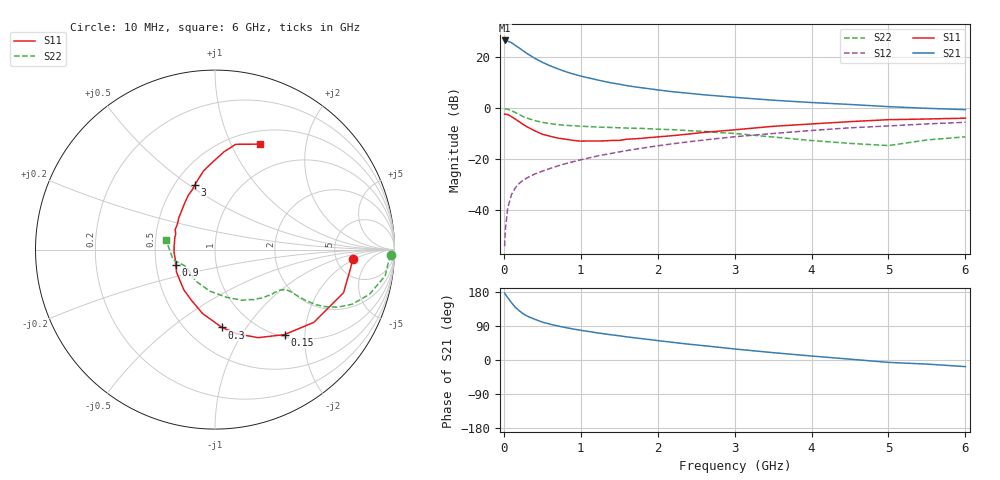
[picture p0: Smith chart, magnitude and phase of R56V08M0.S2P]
! SIEMENS Small Signal Semiconductors
! BFR183
! Si NPN RF Bipolar Junction Transistor in SOT23
! VCE = 6 V  IC = 8 mA
! Common Emitter S-Parameters:  May  1996
# GHz  S  MA  R  50
!  f  S11  S21  S12  S22
! GHz  MAG  ANG  MAG  ANG  MAG  ANG  MAG  ANG
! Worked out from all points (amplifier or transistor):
!   36 points, 10 MHz to 6 GHz, reference 50 ohm
!   highest |S21| = 26.5 dB at 10 MHz (marker M1)
!   |S21| within 3 dB of that: start of sweep to 202.4 MHz
!   unconditionally stable (mu >= 1): 884.2 MHz to 2.593 GHz
!   at 250 MHz: K = 0.54, MSG = 25.4 dB, |S12| = -28.2 dB
!   at 1.4 GHz: K = 1.05, MAG = 12.4 dB, |S12| = -17.7 dB
!   at 6 GHz: K = 0.88, MSG = 2.5 dB, |S12| = -5.5 dB
!   lowest NFmin = 1.30 dB at 450 MHz
!   S11 on the Smith chart (normalised r, x): 10 MHz: 7.21, -1.80; 150 MHz: 1.04, -1.58; 300 MHz: 0.73, -0.78; 900 MHz: 0.63, -0.11; 3 GHz: 0.63, +0.53; 6 GHz: 0.65, +1.30
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0.01  0.7694 -3.8  21.23 176.7  0.002 87.8  0.9827 -1.8
0.02  0.7628 -7.6  20.92 173.4  0.0043 87.5  0.9704 -3.6
0.05  0.7554 -18.5  20.54 164.7  0.011 81.1  0.9591 -8.8
0.1  0.6842 -36.3  19.14 151.0  0.0206 74.0  0.8955 -16.2
0.15  0.6118 -50.7  16.95 139.0  0.0279 67.2  0.8227 -21.7
0.2  0.5464 -63.9  15.12 129.9  0.0339 64.4  0.7533 -25.2
0.25  0.484 -75.6  13.36 122.1  0.0389 62.4  0.6906 -27.4
0.3  0.4353 -84.9  11.83 116.2  0.0433 61.2  0.6418 -28.6
0.4  0.3629 -101.0  9.558 107.6  0.0514 60.9  0.5759 -29.3
0.5  0.3104 -115.3  7.929 100.1  0.0587 61.4  0.53 -29.3
0.6  0.2838 -127.6  6.79 94.6  0.0661 61.8  0.4997 -29.2
0.7  0.261 -138.4  5.931 89.9  0.0743 63.0  0.4798 -29.0
0.9  0.2351 -158.6  4.69 81.9  0.09 62.9  0.4542 -29.4
1.1  0.2289 -175.5  3.934 75.3  0.1062 63.5  0.4377 -30.9
1.3  0.2295 169.3  3.36 69.2  0.1231 63.1  0.4247 -32.3
1.6  0.2481 153.4  2.772 61.0  0.1486 62.0  0.409 -35.7
2.2  0.2913 128.6  2.102 46.5  0.2021 57.9  0.3806 -44.7
3  0.3783 107.3  1.638 29.1  0.2767 50.1  0.3212 -61.6
3.5  0.4433 98.3  1.436 19.4  0.3207 44.3  0.2738 -76.3
4.5  0.5474 84.7  1.187 2.2  0.4144 32.4  0.2054 -121.9
5.5  0.6167 72.1  0.997 -10.8  0.4939 20.6  0.2399 -166.4
6  0.6392 66.9  0.941 -17.4  0.5314 12.8  0.2762 169.4
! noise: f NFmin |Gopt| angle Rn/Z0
0.45  1.3  0.17  43  0.21
0.9  1.35  0.21  115  0.2
1.8  2.05  0.33  -177  0.14
